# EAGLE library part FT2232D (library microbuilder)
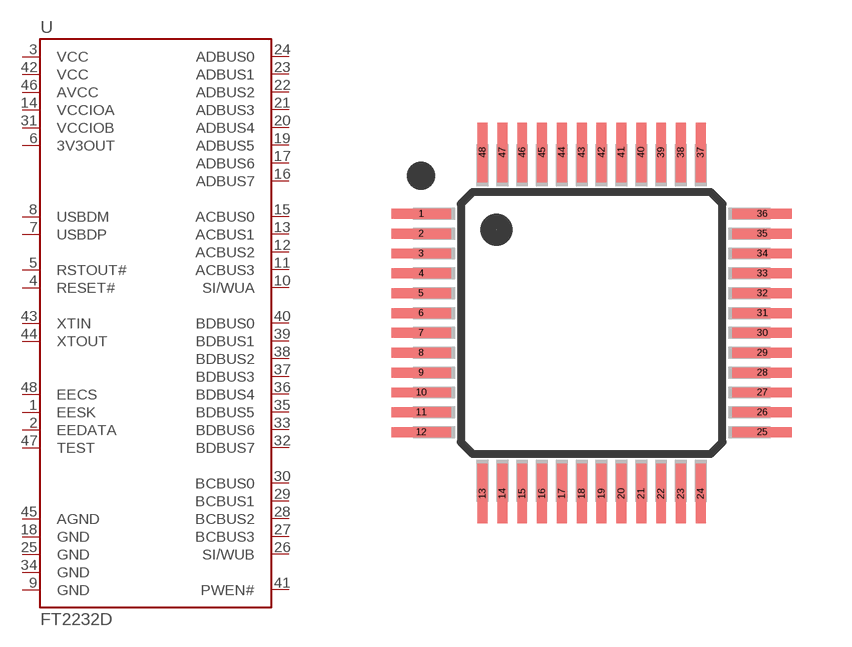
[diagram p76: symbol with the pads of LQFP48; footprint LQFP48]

Designator prefix -

## FT2232D  [LQFP48]
1  EESK
2  EEDATA
3  VCC  pwr
4  RESET#
5  RSTOUT#
6  3V3OUT  pwr
7  USBDP
8  USBDM
9  GND  pwr
10  SI/WUA
11  ACBUS3
12  ACBUS2
13  ACBUS1
14  VCCIOA  pwr
15  ACBUS0
16  ADBUS7
17  ADBUS6
18  GND  pwr
19  ADBUS5
20  ADBUS4
21  ADBUS3
22  ADBUS2
23  ADBUS1
24  ADBUS0
25  GND  pwr
26  SI/WUB
27  BCBUS3
28  BCBUS2
29  BCBUS1
30  BCBUS0
31  VCCIOB  pwr
32  BDBUS7  in
33  BDBUS6  in
34  GND  pwr
35  BDBUS5  in
36  BDBUS4  out
37  BDBUS3  in
38  BDBUS2  out
39  BDBUS1  in
40  BDBUS0  out
41  PWEN#
42  VCC  pwr
43  XTIN
44  XTOUT
45  AGND  pwr
46  AVCC  pwr
47  TEST  in
48  EECS

## Footprint LQFP48 (pad centres in mm)
smd 1.5 x 0.25: 1 -4.3,2.75; 2 -4.3,2.25; 3 -4.3,1.75; 4 -4.3,1.25; 5 -4.3,0.75; 6 -4.3,0.25; 7 -4.3,-0.25; 8 -4.3,-0.75; 9 -4.3,-1.25; 10 -4.3,-1.75; 11 -4.3,-2.25; 12 -4.3,-2.75; 25 4.3,-2.75; 26 4.3,-2.25; 27 4.3,-1.75; 28 4.3,-1.25; 29 4.3,-0.75; 30 4.3,-0.25; 31 4.3,0.25; 32 4.3,0.75; 33 4.3,1.25; 34 4.3,1.75; 35 4.3,2.25; 36 4.3,2.75
smd 0.25 x 1.5: 13 -2.75,-4.3; 14 -2.25,-4.3; 15 -1.75,-4.3; 16 -1.25,-4.3; 17 -0.75,-4.3; 18 -0.25,-4.3; 19 0.25,-4.3; 20 0.75,-4.3; 21 1.25,-4.3; 22 1.75,-4.3; 23 2.25,-4.3; 24 2.75,-4.3; 37 2.75,4.3; 38 2.25,4.3; 39 1.75,4.3; 40 1.25,4.3; 41 0.75,4.3; 42 0.25,4.3; 43 -0.25,4.3; 44 -0.75,4.3; 45 -1.25,4.3; 46 -1.75,4.3; 47 -2.25,4.3; 48 -2.75,4.3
